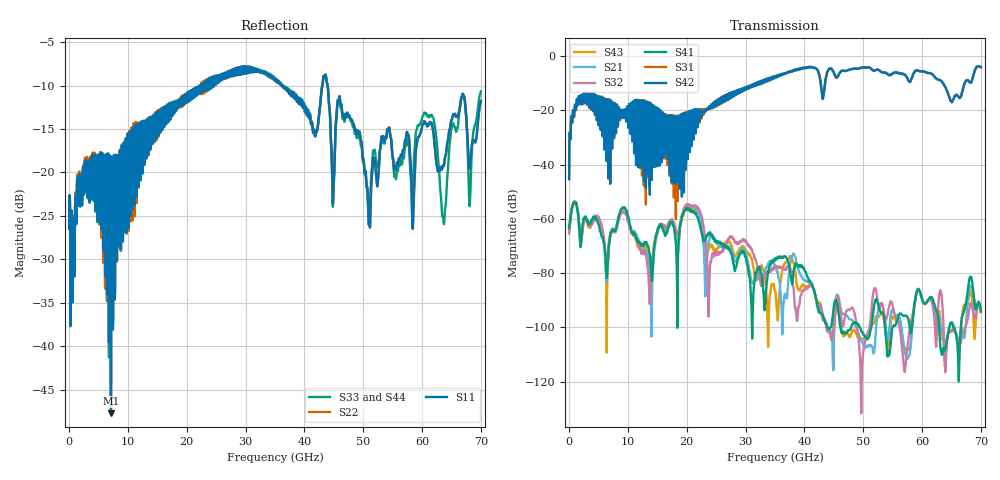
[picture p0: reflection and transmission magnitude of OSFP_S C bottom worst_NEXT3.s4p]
! AWR Design Environment (8415) Mon Jan 07 17:44:51 2019
! Document = 'OSFP Channel_S'
! nPorts: 4, nXvals: 7001
# HZ S DB R 50
!Freq DBS11 AngS11 DBS12 AngS12 DBS13 AngS13 DBS14 AngS14
!	DBS21 AngS21 DBS22 AngS22 DBS23 AngS23 DBS24 AngS24
!	DBS31 AngS31 DBS32 AngS32 DBS33 AngS33 DBS34 AngS34
!	DBS41 AngS41 DBS42 AngS42 DBS43 AngS43 DBS44 AngS44
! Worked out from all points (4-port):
!   7000 points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, 10 MHz to 70 GHz, reference 50 ohm
!   strongest paths, dB at 10 MHz, 17.51 GHz, 35.01 GHz, 52.51 GHz, 70 GHz:
!     S42: -45.3, -29.4, -7.4, -4.9, -4.0
!     S31: -45.4, -29.5, -7.4, -4.9, -4.0
!     S41: -63.4, -61.1, -75.1, -91.4, -94.1
!     S32: -65.4, -60.1, -78.2, -91.2, -93.9
!     S21: -64.1, -60.7, -77.4, -94.0, -93.6
!     S43: -63.6, -60.4, -86.5, -96.3, -94.5
!   lowest |S11| = -47.7 dB at 7.12 GHz (marker M1), VSWR 1.01, Z = 50.1 - j0.408 ohm
!   |S11| at or under -10 dB: start of sweep to 22.43 GHz; 36.33 GHz to 43.05 GHz (6.718 GHz wide, 16.9 % of centre); 43.97 GHz to end of sweep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
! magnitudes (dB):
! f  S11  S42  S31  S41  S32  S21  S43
! 10 MHz  -26.5  -45.3  -45.4  -63.4  -65.4  -64.1  -63.6
! 1.65 GHz  -21.1  -14.7  -14.8  -61.6  -59.9  -60.9  -60.5
! 7.12 GHz  -47.7  -16.7  -16.7  -65.1  -64.8  -64.4  -65.4
! 13.95 GHz  -14.2  -19.3  -19.3  -78.3  -80.1  -90.6  -84.1
! 20.21 GHz  -11.5  -33.8  -33.5  -56.0  -54.4  -54.7  -55.6
! 23.8 GHz  -9.2  -18.5  -18.7  -65.7  -87.8  -68.2  -70.9
! 70 GHz  -11.8  -4.0  -4.0  -94.1  -93.9  -93.6  -94.5
